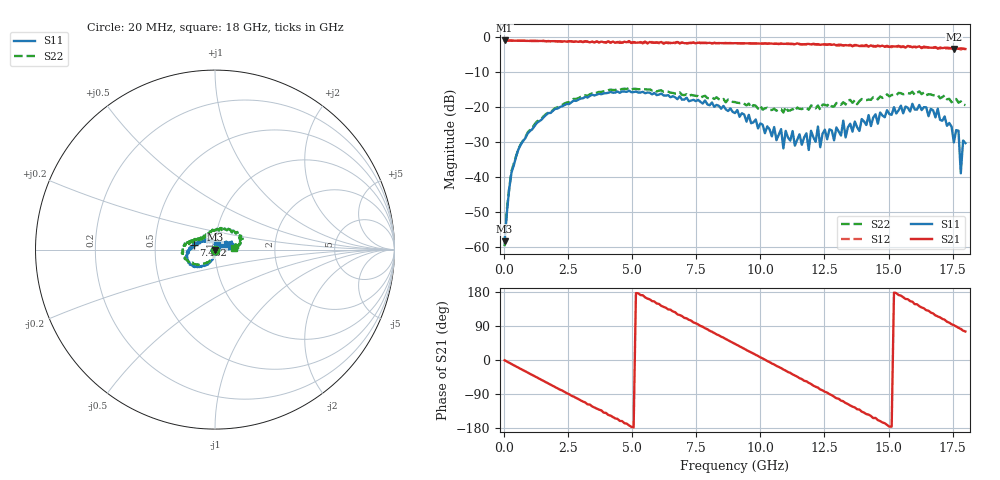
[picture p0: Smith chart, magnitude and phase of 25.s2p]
!Agilent Technologies,N5230A,US43500223,A.07.50.48
!Agilent N5230A: A.07.50.48
!Date: Sunday, January 31, 2016 11:28:40
!Correction: S11(Full 2 Port(1,2))
!S21(Full 2 Port(1,2))
!S12(Full 2 Port(1,2))
!S22(Full 2 Port(1,2))
!S2P File: Measurements: S11, S21, S12, S22:
# Hz S  RI  R 50
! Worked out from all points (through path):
!   201 points, 20 MHz to 18 GHz, reference 50 ohm
!   highest |S21| = -1.01 dB at 20 MHz (marker M1); lowest = -3.5 dB at 17.55 GHz (marker M2)
!   group delay of S21, straight-line fit = 99 ps
!   lowest |S11| = -58.4 dB at 20 MHz (marker M3), VSWR 1.00, Z = 50 - j0.118 ohm
!   |S11| at or under -10 dB: start of sweep to end of sweep
!   |S22| runs from -59.8 to -14.6 dB; largest |S21 - S12| = 0.068
!   S11 on the Smith chart (normalised r, x): 20 MHz: 1.00, -0.00; 7.482 GHz: 0.79, +0.04; 18 GHz: 1.02, +0.06
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2e7  -0.000227 -0.00118  0.8898 -0.0124  0.8909 -0.0152  -0.00101 9.21e-05
2.897e8  0.00177 -0.0114  0.8701 -0.1636  0.8707 -0.1646  0.00135 -0.0121
6.493e8  0.000836 -0.0288  0.8087 -0.3526  0.808 -0.3536  -0.00239 -0.0291
1.9978e9  -0.0408 -0.0845  0.276 -0.8252  0.2642 -0.8289  -0.0582 -0.0769
3.0766e9  -0.0927 -0.0951  -0.2841 -0.7928  -0.2958 -0.7971  -0.1155 -0.0801
4.515e9  -0.1436 -0.0673  -0.777 -0.2721  -0.8104 -0.2711  -0.1712 -0.0329
6.0433e9  -0.1499 -0.00651  -0.701 0.4388  -0.6726 0.4529  -0.1691 0.0214
7.4817e9  -0.1179 0.0263  -0.0983 0.8032  -0.0736 0.8109  -0.1383 0.04
9.01e9  -0.0629 0.0518  0.6016 0.5496  0.6186 0.5311  -0.1037 0.0547
1.04484e10  0.00301 0.0377  0.7943 -0.1276  0.7873 -0.1546  -0.0654 0.062
1.08979e10  0.00587 0.0248  0.7216 -0.3369  0.7136 -0.3627  -0.054 0.063
1.17969e10  0.0141 0.0395  0.4408 -0.6577  0.3914 -0.6792  -0.0357 0.09
1.18868e10  0.0174 0.0169  0.3952 -0.6901  0.3533 -0.6982  -0.0345 0.0843
1.20666e10  0.0154 0.0334  0.3028 -0.7394  0.2791 -0.7386  -0.0284 0.0983
1.36848e10  0.0566 0.0244  -0.442 -0.6292  -0.4546 -0.6025  0.0314 0.1204
1.50333e10  0.0666 0.0427  -0.7164 -0.0537  -0.725 -0.0192  0.0967 0.1026
1.69212e10  0.0938 0.0069  -0.2894 0.6149  -0.2463 0.6501  0.1436 0.0349
1.75505e10  0.0303 0.00674  -0.0209 0.6707  0.0255 0.6752  0.124 0.0246
1.77303e10  0.0416 0.0188  0.0609 0.6734  0.1044 0.6708  0.1133 0.019
1.78202e10  0.0112 -0.000827  0.094 0.6816  0.1388 0.6497  0.1161 0.0297
1.79101e10  0.0303 0.0132  0.1479 0.6658  0.1803 0.6517  0.1075 0.017
1.8e10  0.0121 0.0278  0.1716 0.6507  0.2262 0.6277  0.1053 0.00989
